ORGANIZATION_BLOCK OB 1
BEGIN

	// Start timer and let it expire
	__STWRST
	L		0
	SA		T 10
	SET
	R		T 10
	U		T 10
	__ASSERT==	__STW VKE,	0
	SET
	L		W#16#0010
	SA		T 10
	U		T 10
	__ASSERT==	__STW VKE,	1
	L		T 10
	__ASSERT==	__ACCU 1,	0
	__SLEEP		101
	U		T 10
	__ASSERT==	__STW VKE,	1
	L		T 10
	__ASSERT==	__ACCU 1,	0


	// Start timer and reset VKE
	__STWRST
	L		0
	SA		T 10
	SET
	R		T 10
	U		T 10
	__ASSERT==	__STW VKE,	0
	SET
	L		W#16#0010
	SA		T 10
	U		T 10
	__ASSERT==	__STW VKE,	1
	L		T 10
	__ASSERT==	__ACCU 1,	0
	__SLEEP		101
	L		T 10
	__ASSERT==	__ACCU 1,	0
	CLR
	L		W#16#0010
	SA		T 10
	U		T 10
	__ASSERT==	__STW VKE,	1
	L		T 10
	__ASSERT>=	__ACCU 1,	5
	__SLEEP		101
	U		T 10
	__ASSERT==	__STW VKE,	0
	L		T 10
	__ASSERT==	__ACCU 1,	0


	// Retrigger
	__STWRST
	L		0
	SA		T 10
	SET
	R		T 10
	U		T 10
	__ASSERT==	__STW VKE,	0
	SET
	L		W#16#0010
	SA		T 10
	U		T 10
	__ASSERT==	__STW VKE,	1
	L		T 10
	__ASSERT==	__ACCU 1,	0
	CLR
	L		W#16#0010
	SA		T 10
	__SLEEP		20
	SET
	SA		T 10
	L		T 10
	__ASSERT>=	__ACCU 1,	2
	__SLEEP		101
	L		T 10
	__ASSERT==	__ACCU 1,	__ACCU 2


	// Reset signal
	__STWRST
	L		0
	SA		T 10
	SET
	R		T 10
	U		T 10
	__ASSERT==	__STW VKE,	0
	SET
	L		W#16#0010
	SA		T 10
	U		T 10
	__ASSERT==	__STW VKE,	1
	L		T 10
	__ASSERT==	__ACCU 1,	0
	__ASSERT==	__ACCU 1,	0
	CLR
	L		W#16#0010
	SA		T 10
	U		T 10
	__ASSERT==	__STW VKE,	1
	L		T 10
	__ASSERT>=	__ACCU 1,	5
	SET
	R		T 10
	U		T 10
	__ASSERT==	__STW VKE,	0
	L		T 10
	__ASSERT==	__ACCU 1,	0
	__SLEEP		101
	U		T 10
	__ASSERT==	__STW VKE,	0
	L		T 10
	__ASSERT==	__ACCU 1,	0


	// Test timer parameter
	AUF		DB 1
	L		DBW 0
	__ASSERT==	__ACCU 1,	24
	CALL FB 1, DB 1 (
		TIMER_VAR	:= T 42
	)
END_ORGANIZATION_BLOCK


FUNCTION_BLOCK FB 1
	VAR_INPUT
		TIMER_VAR	: TIMER
	END_VAR
BEGIN
	L		DIW 0
	__ASSERT==	__ACCU 1,	42
	L		#TIMER_VAR
	__ASSERT==	__ACCU 1,	0
	U		#TIMER_VAR
	__ASSERT==	__STW VKE,	0

	SA		#TIMER_VAR
END_FUNCTION_BLOCK


DATA_BLOCK DB 1
	FB 1
BEGIN
	TIMER_VAR	:= T 24
END_DATA_BLOCK
